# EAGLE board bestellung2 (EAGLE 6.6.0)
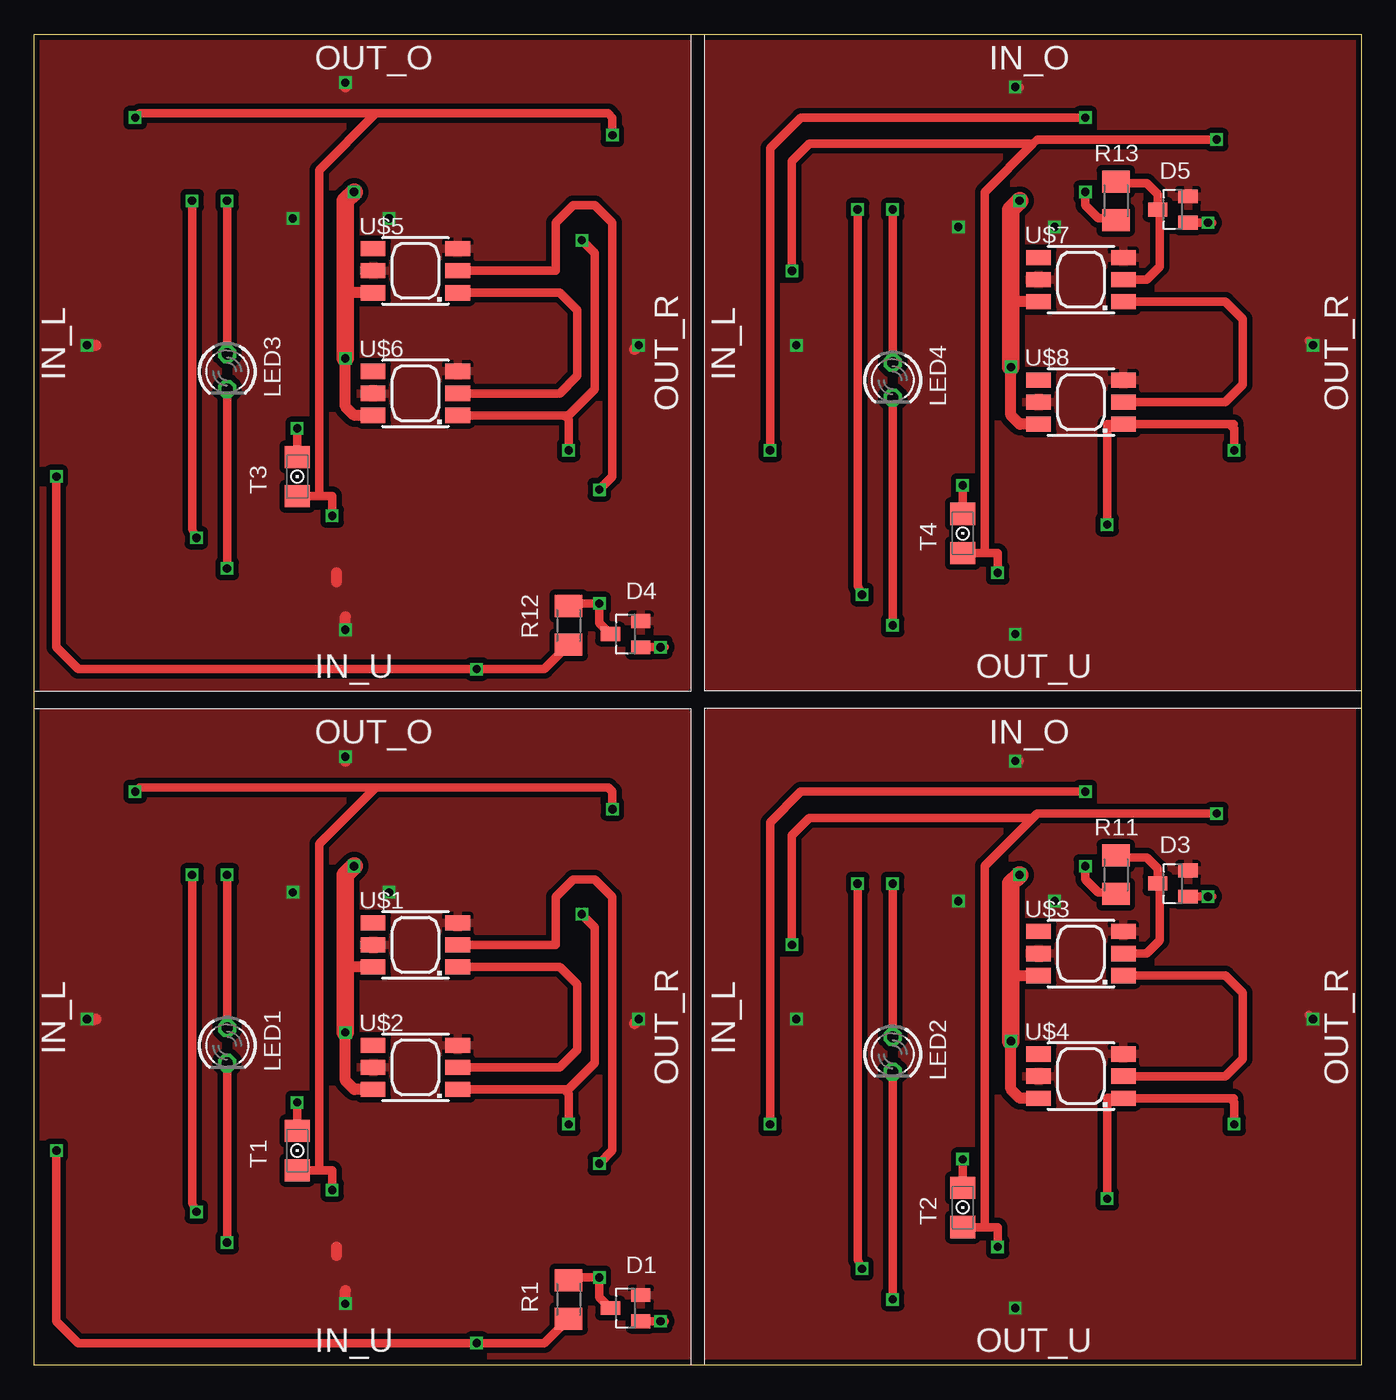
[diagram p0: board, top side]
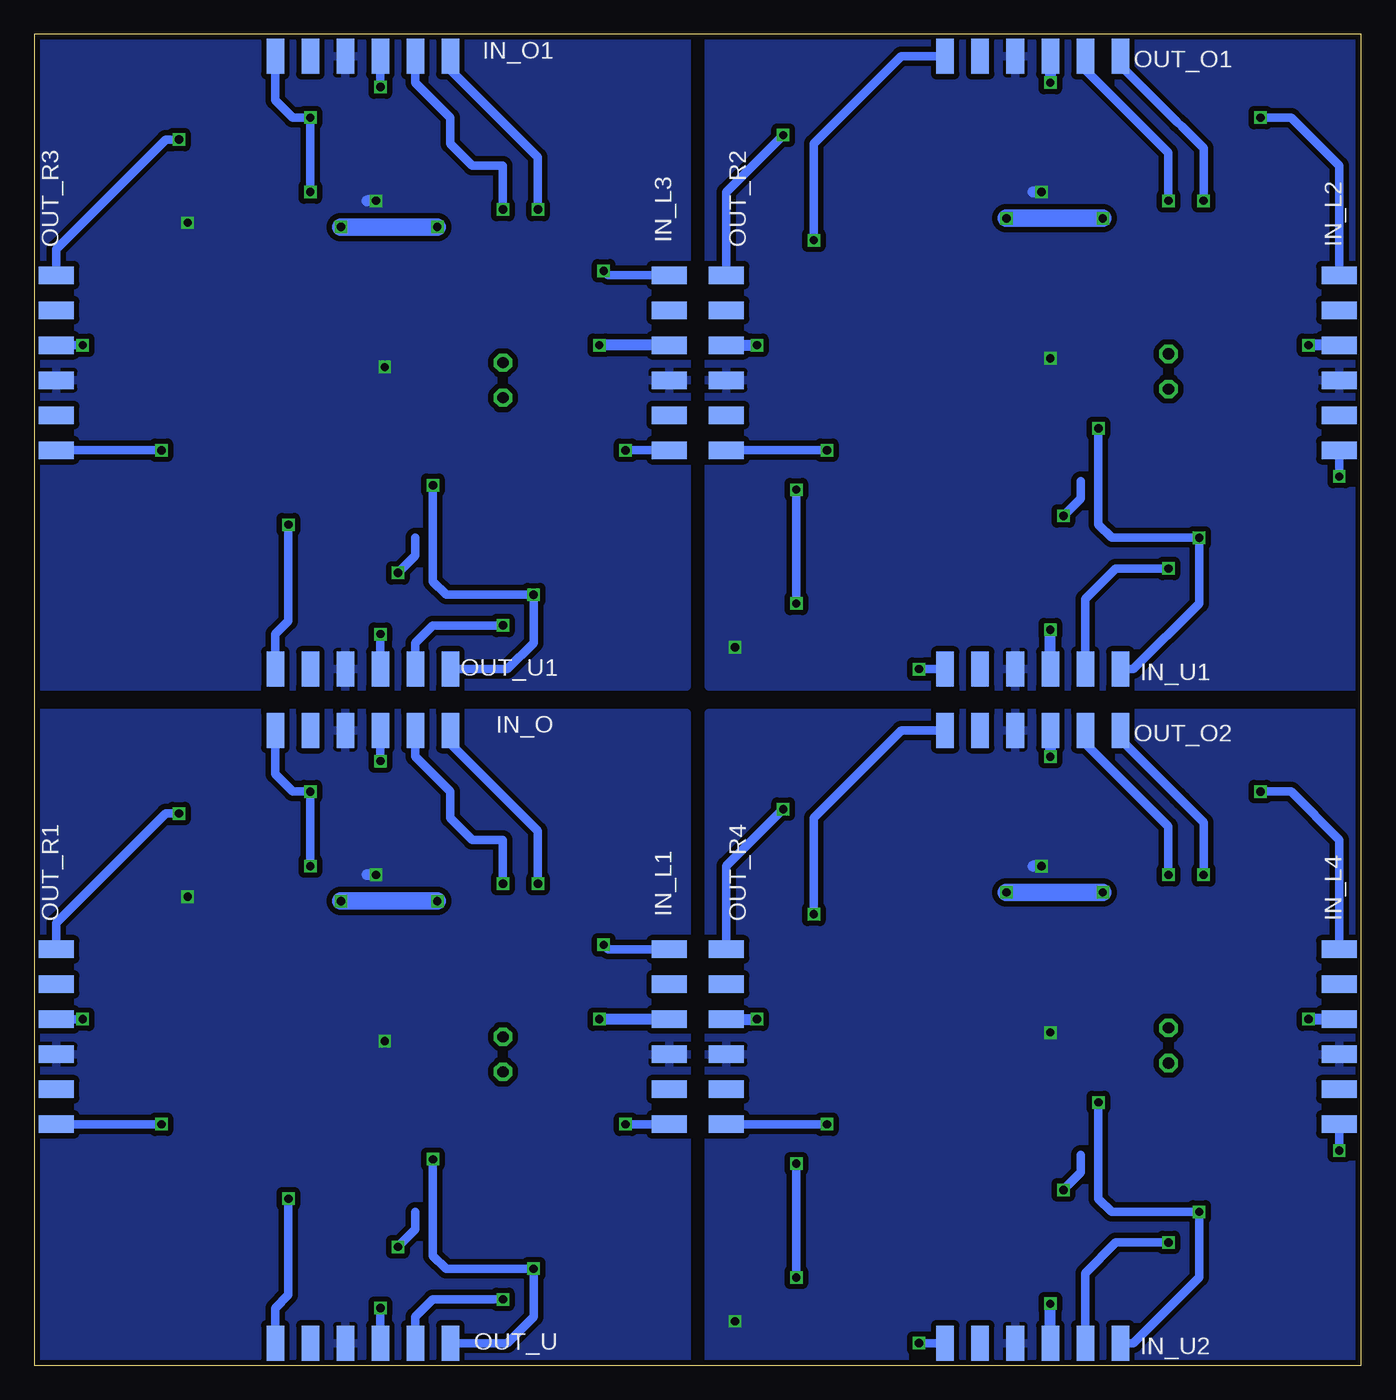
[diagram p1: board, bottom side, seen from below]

Size 96.2 x 96.52 mm. Coordinates in mm from the lower left corner, seen from the top.
Outline: 0,0 0,96.52 96.2,96.52 96.2,0 0,0
Copper layers (1*16): Top 0.035mm / dielectric 1.5mm / Bottom 0.035mm
Design rules "Elecrow_2-layer_eagle_rule": minimum track width 6mil, minimum drill 12mil, track to track 6mil, track to pad 6mil, pad to pad 6mil, via to via 6mil, smd to smd 0mil, copper to edge 10mil, drill to drill 10mil, minimum pad ring 10mil, minimum via ring 6mil, stop-mask expansion 2mil, vias tented up to drill 100mil, thermal gap 10mil

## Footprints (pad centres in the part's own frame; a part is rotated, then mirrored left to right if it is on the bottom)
SOT23 = smd 1 x 1.4: 1 -0.95,-1.1; 2 0.95,-1.1; 3 0,1.1
SMD1,27-2,54-6 = smd 1.27 x 2.54: 1 0,0; 2 2.54,0; 3 5.08,0; 4 7.62,0; 5 10.16,0; 6 12.7,0
LED3MM = drill 0.813 octagon: A -1.27,0; K 1.27,0
M1206 = smd 1.6 x 2: 1 -1.4,0; 2 1.4,0
1206 = smd 1.6 x 1.803: A -1.422,0; C 1.422,0
CLN6A = smd 1.778 x 1.1: 1 3.071,-1.6; 2 3.071,0; 3 3.071,1.6; 4 -3.071,1.6; 5 -3.071,0; 6 -3.071,-1.6

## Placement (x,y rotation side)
D1  BAS40-04  [SOT23]  42.86,4.13 90 top
D3  BAS40-04  [SOT23]  82.55,34.92 90 top
D4  BAS40-04  [SOT23]  42.86,53.02 90 top
D5  BAS40-04  [SOT23]  82.55,83.82 90 top
IN_L1  SMD2-6  [SMD1,27-2,54-6]  50.16,30.16 270 bottom
IN_L2  SMD2-6  [SMD1,27-2,54-6]  1.59,79.06 270 bottom
IN_L3  SMD2-6  [SMD1,27-2,54-6]  50.16,79.06 270 bottom
IN_L4  SMD2-6  [SMD1,27-2,54-6]  1.59,30.16 270 bottom
IN_O  SMD2-6  [SMD1,27-2,54-6]  66.04,46.04 180 bottom
IN_O1  SMD2-6  [SMD1,27-2,54-6]  66.04,94.93 180 bottom
IN_U1  SMD2-6  [SMD1,27-2,54-6]  17.46,50.48 180 bottom
IN_U2  SMD2-6  [SMD1,27-2,54-6]  17.46,1.59 180 bottom
LED1  [LED3MM]  13.97,23.18 270 top
LED2  [LED3MM]  62.23,22.54 270 top
LED3  [LED3MM]  13.97,72.07 270 top
LED4  [LED3MM]  62.23,71.44 270 top
OUT_O1  SMD2-6  [SMD1,27-2,54-6]  17.46,94.93 180 bottom
OUT_O2  SMD2-6  [SMD1,27-2,54-6]  17.46,46.04 180 bottom
OUT_R1  SMD2-6  [SMD1,27-2,54-6]  94.61,30.16 270 bottom
OUT_R2  SMD2-6  [SMD1,27-2,54-6]  46.04,79.06 270 bottom
OUT_R3  SMD2-6  [SMD1,27-2,54-6]  94.61,79.06 270 bottom
OUT_R4  SMD2-6  [SMD1,27-2,54-6]  46.04,30.16 270 bottom
OUT_U  SMD2-6  [SMD1,27-2,54-6]  66.04,1.59 180 bottom
OUT_U1  SMD2-6  [SMD1,27-2,54-6]  66.04,50.48 180 bottom
R1  [M1206]  38.73,4.76 90 top
R11  [M1206]  78.42,35.56 90 top
R12  [M1206]  38.73,53.66 90 top
R13  [M1206]  78.42,84.45 90 top
T1  PHOTO-TRANS-1206  [1206]  19.05,15.56 90 top
T2  PHOTO-TRANS-1206  [1206]  67.31,11.43 90 top
T3  PHOTO-TRANS-1206  [1206]  19.05,64.45 90 top
T4  PHOTO-TRANS-1206  [1206]  67.31,60.33 90 top
U$1  LED_SMD5050  [CLN6A]  27.62,30.48 0 top
U$2  LED_SMD5050  [CLN6A]  27.62,21.59 0 top
U$3  LED_SMD5050  [CLN6A]  75.88,29.84 0 top
U$4  LED_SMD5050  [CLN6A]  75.88,20.95 0 top
U$5  LED_SMD5050  [CLN6A]  27.62,79.38 0 top
U$6  LED_SMD5050  [CLN6A]  27.62,70.48 0 top
U$7  LED_SMD5050  [CLN6A]  75.88,78.74 0 top
U$8  LED_SMD5050  [CLN6A]  75.88,69.85 0 top

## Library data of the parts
D1 D3-D5 = diode
IN_L1-IN_L4 IN_O IN_O1 IN_U1 IN_U2 OUT_O1 OUT_O2 OUT_R1-OUT_R4 OUT_U OUT_U1 T1-T4 U$1-U$8 = #mylib
LED1-LED4 = led
R1 R11-R13 = resistor

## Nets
+5V1: D3.2 IN_L1.3 IN_O.3 OUT_R1.3 OUT_U.3 U$3.3 U$3.5 U$4.3 U$4.5
+5V2: D4.2 IN_L2.3 IN_U1.3 OUT_O1.3 OUT_R2.3 U$5.3 U$5.5 U$6.3 U$6.5
+5V3: D5.2 IN_L3.3 IN_O1.3 OUT_R3.3 OUT_U1.3 U$7.3 U$7.5 U$8.3 U$8.5
+5V4: D1.2 IN_L4.3 IN_U2.3 OUT_O2.3 OUT_R4.3 U$1.3 U$1.5 U$2.3 U$2.5
GND1: D3.1 IN_L1.4 IN_O.4 OUT_R1.4 OUT_U.4 U$3.6 U$4.6
GND2: D4.1 IN_L2.4 IN_U1.4 OUT_O1.4 OUT_R2.4 U$5.6 U$6.6
GND3: D5.1 IN_L3.4 IN_O1.4 OUT_R3.4 OUT_U1.4 U$7.6 U$8.6
GND4: D1.1 IN_L4.4 IN_U2.4 OUT_O2.4 OUT_R4.4 U$1.6 U$2.6
N$1: U$1.1 U$2.2
N$2: IN_U2.1 OUT_O2.1 T1.C
N$3: LED1.A OUT_O2.2
N$4: IN_U2.2 LED1.K
N$5: IN_L4.6 IN_U2.6 R1.1
N$6: IN_L4.1 OUT_R4.1 T1.A
N$7: D1.3 R1.2 U$1.2
N$8: OUT_O2.6 OUT_R4.6 U$2.1
N$12: U$3.1 U$4.2
N$16: IN_O.1 OUT_U.1 T2.C
N$20: IN_O.2 LED2.A
N$22: LED2.K OUT_U.2
N$23: IN_L1.6 IN_O.6 R11.1
N$24: IN_L1.1 OUT_R1.1 T2.A
N$26: D3.3 R11.2 U$3.2
N$27: OUT_R1.6 OUT_U.6 U$4.1
N$28: U$5.1 U$6.2
N$29: IN_U1.1 OUT_O1.1 T3.C
N$30: LED3.A OUT_O1.2
N$31: IN_U1.2 LED3.K
N$32: IN_L2.6 IN_U1.6 R12.1
N$33: IN_L2.1 OUT_R2.1 T3.A
N$34: D4.3 R12.2 U$5.2
N$35: OUT_O1.6 OUT_R2.6 U$6.1
N$36: U$7.1 U$8.2
N$37: IN_O1.1 OUT_U1.1 T4.C
N$38: IN_O1.2 LED4.A
N$39: LED4.K OUT_U1.2
N$40: IN_L3.6 IN_O1.6 R13.1
N$41: IN_L3.1 OUT_R3.1 T4.A
N$42: D5.3 R13.2 U$7.2
N$43: OUT_R3.6 OUT_U1.6 U$8.1

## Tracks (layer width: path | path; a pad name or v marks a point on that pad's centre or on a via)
+5V1  (via drill 0.6)
  Top 0.61: v71.12,43.81 71.44,43.81 | v92.71,25.08 92.39,25.4
  Bottom 0.61: IN_O.3 v71.12,43.81 | OUT_R1.3 v92.71,25.08 | v71.12,4.13 OUT_U.3
  Bottom 0.813: IN_L1.3 v55.24,25.08
  Bottom 1.27: v66.99,33.66 v73.98,33.66
  pour Top (isolate 0.406): 48.9,47.31 95.89,47.31 95.89,0.32 48.9,0.32
+5V2  (via drill 0.6)
  Top 0.813: 21.91,56.83 21.91,57.47 | v43.81,73.98 43.5,73.66 | v22.54,53.34 22.54,54.29 | v3.81,73.98 4.45,73.98 | v22.54,93.03 22.54,92.71
  Bottom 0.813: OUT_R2.3 v43.81,73.98 | IN_U1.3 v22.54,53.34 | IN_L2.3 v3.81,73.98 | OUT_O1.3 v22.54,93.03
  Bottom 1.27: v18.73,83.19 v25.72,83.19
  pour Top (isolate 0.406): 0.32,96.2 47.31,96.2 47.31,49.21 0.32,49.21
+5V3  (via drill 0.6)
  Top 0.61: v71.12,92.71 71.44,92.71 | v92.71,73.98 92.39,74.3
  Bottom 0.61: IN_O1.3 v71.12,92.71 | OUT_R3.3 v92.71,73.98 | v71.12,53.02 OUT_U1.3
  Bottom 0.813: IN_L3.3 v55.24,73.98
  Bottom 1.27: v66.99,82.55 v73.98,82.55
  pour Top (isolate 0.406): 48.9,96.2 95.89,96.2 95.89,49.21 48.9,49.21
+5V4  (via drill 0.6)
  Top 0.813: 21.91,7.94 21.91,8.57 | v43.81,25.08 43.5,24.77 | v22.54,4.45 22.54,5.4 | v3.81,25.08 4.45,25.08 | v22.54,44.13 22.54,43.81
  Bottom 0.813: OUT_R4.3 v43.81,25.08 | IN_U2.3 v22.54,4.45 | IN_L4.3 v3.81,25.08 | OUT_O2.3 v22.54,44.13
  Bottom 1.27: v18.73,34.29 v25.72,34.29
  pour Top (isolate 0.406): 0.32,47.31 47.31,47.31 47.31,0.32 0.32,0.32
GND1  (via drill 0.6)
  Top 0.61: D3.1 85.41,33.98 v85.09,33.97
  Top 0.813: U$4.6 71.45,19.36 70.8,20 v70.8,23.5 | U$3.6 70.81,28.25 70.8,28.26
  Top 1.27: v70.8,23.5 70.8,28.26 70.8,34.92 v71.44,35.56
  Bottom 0.813: v71.44,35.56 72.07,35.56
  pour Bottom (isolate 0.406): 48.9,47.31 95.89,47.31 95.89,0.32 48.9,0.32
GND2  (via drill 0.6)
  Top 0.61: D4.1 45.72,52.07 v45.4,52.07
  Top 0.813: U$6.6 23.19,68.89 22.54,69.53 v22.54,73.03 | U$5.6 22.55,77.78 22.54,77.79
  Top 1.27: v22.54,73.03 22.54,77.79 22.54,84.45 v23.18,85.09
  Bottom 0.813: v23.18,85.09 23.81,85.09
  pour Bottom (isolate 0.406): 0.32,96.2 47.31,96.2 47.31,49.21 0.32,49.21
GND3  (via drill 0.6)
  Top 0.61: D5.1 85.41,82.87 v85.09,82.87
  Top 0.813: U$8.6 71.45,68.25 70.8,68.9 v70.8,72.39 | U$7.6 70.81,77.14 70.8,77.15
  Top 1.27: v70.8,72.39 70.8,77.15 70.8,83.82 v71.44,84.45
  Bottom 0.813: v71.44,84.45 72.07,84.45
  pour Bottom (isolate 0.406): 48.9,96.2 95.89,96.2 95.89,49.21 48.9,49.21
GND4  (via drill 0.6)
  Top 0.61: D1.1 45.72,3.18 v45.4,3.17
  Top 0.813: U$2.6 23.19,19.99 22.54,20.64 v22.54,24.13 | U$1.6 22.55,28.88 22.54,28.89
  Top 1.27: v22.54,24.13 22.54,28.89 22.54,35.56 v23.18,36.2
  Bottom 0.813: v23.18,36.2 23.81,36.2
  pour Bottom (isolate 0.406): 0.32,47.31 47.31,47.31 47.31,0.32 0.32,0.32
N$1
  Top 0.61: U$2.2 38.1,21.59 39.37,22.86 39.37,27.62 38.1,28.89 30.71,28.89 U$1.1
N$2  (via drill 0.6)
  Top 0.61: v11.43,35.56 11.43,11.75 v11.75,11.11 | v19.05,19.05 T1.C
  Bottom 0.61: v11.43,35.56 11.43,39.37 13.02,40.96 13.34,41.27 17.46,45.4 OUT_O2.1 | v19.05,19.05 19.05,12.06 18.1,11.11 v11.75,11.11 11.75,6.35 16.51,1.59 IN_U2.1
N$3  (via drill 0.6)
  Top 0.61: v13.97,35.56 LED1.A
  Bottom 0.61: v13.97,35.56 13.97,39.05 20,45.09 OUT_O2.2
N$4  (via drill 0.6)
  Top 0.61: v13.97,8.89 LED1.K
  Bottom 0.61: v13.97,8.89 17.78,8.89 20,6.67 IN_U2.2
N$5  (via drill 0.6)
  Top 0.61: R1.1 36.96,1.59 v32.07,1.59 3.17,1.59 1.59,3.17 v1.59,15.56
  Bottom 0.61: IN_U2.6 v32.07,1.59 | IN_L4.6 v1.59,15.56
N$6  (via drill 0.6)
  Top 0.61: v21.59,12.7 21.59,14.14 T1.A 20.64,14.14 20.64,37.78 24.77,41.91 | v41.91,40.32 41.91,41.59 41.59,41.91 24.77,41.91 | v7.3,41.59 7.62,41.91 24.77,41.91
  Bottom 0.61: 20.32,15.24 20.32,13.97 v21.59,12.7 | OUT_R4.1 46.04,36.2 v41.91,40.32 | v7.3,41.59 5.08,41.59 1.59,38.1 IN_L4.1
N$7  (via drill 0.6)
  Top 0.61: 41.91,3.98 D1.3 40.96,4.93 v40.96,6.35 38.92,6.35 R1.2 | U$1.2 37.78,30.48 37.78,33.97 39.05,35.24 40.64,35.24 41.91,33.97 41.91,15.56 v40.96,14.61
  Bottom 0.61: v40.96,6.35 v40.96,14.61
N$8  (via drill 0.6)
  Top 0.61: U$2.1 38.42,19.99 | 38.42,19.99 38.72,19.99 40.64,21.91 40.64,31.75 v39.69,32.7 | v38.73,17.46 38.73,19.67 38.42,19.99
  Bottom 0.61: v39.69,32.7 39.69,39.69 33.34,46.04 OUT_O2.6 | OUT_R4.6 v38.73,17.46
N$12
  Top 0.61: U$4.2 86.36,20.95 87.63,22.23 87.63,26.99 86.36,28.26 78.97,28.26 U$3.1
N$16  (via drill 0.6)
  Top 0.61: v59.69,34.92 59.69,7.62 v60.01,6.99 | v67.31,14.92 T2.C
  Bottom 0.61: v59.69,34.92 59.69,38.73 66.04,45.09 IN_O.1 | v67.31,14.92 67.31,7.94 66.36,6.99 v60.01,6.99 60.01,3.49 61.91,1.59 OUT_U.1
N$20  (via drill 0.6)
  Top 0.61: v62.23,34.92 LED2.A
  Bottom 0.61: v62.23,34.92 62.23,38.1 64.45,38.1 66.04,39.69 66.04,41.59 68.58,44.13 IN_O.2
N$22  (via drill 0.6)
  Top 0.61: v62.23,4.76 LED2.K
  Bottom 0.61: OUT_U.2 68.58,3.49 67.31,4.76 v62.23,4.76
N$23  (via drill 0.6)
  Top 0.61: v76.2,36.2 76.2,35.24 77.15,34.29 78.29,34.29 R11.1 | v53.34,17.46 53.34,39.37 55.56,41.59 v76.2,41.59
  Bottom 0.61: v76.2,36.2 v76.2,41.59 77.47,41.59 78.74,42.86 IN_O.6 | IN_L1.6 v53.34,17.46
N$24  (via drill 0.6)
  Top 0.61: v69.85,8.57 69.85,10.01 68.9,10.01 | 72.39,39.69 72.71,40.01 v85.72,40.01 | 72.39,39.69 68.9,36.2 68.9,10.01 | 68.9,10.01 T2.A | v54.93,30.48 54.93,38.42 56.2,39.69 72.39,39.69
  Bottom 0.61: 68.58,11.11 68.58,9.84 v69.85,8.57 | v85.72,40.01 86.68,40.01 94.61,32.07 OUT_R1.1 | IN_L1.1 54.61,30.16 v54.93,30.48
N$26
  Top 0.61: U$3.2 80.64,29.84 81.6,30.8 81.6,34.78 D3.3 81.45,36.02 80.64,36.83 78.55,36.83 R11.2
N$27  (via drill 0.6)
  Top 0.61: 86.68,19.36 U$4.1 78.95,19.37 77.79,19.37 v77.79,12.06 | 86.68,19.36 86.98,19.36 | v87,17.46 87,19.04 86.68,19.36
  Bottom 0.61: OUT_R1.6 v87,17.46 | v77.79,12.06 77.79,5.08 78.74,4.13 OUT_U.6
N$28
  Top 0.61: U$6.2 38.1,70.48 39.37,71.75 39.37,76.52 38.1,77.79 30.71,77.79 U$5.1
N$29  (via drill 0.6)
  Top 0.61: v11.43,84.45 11.43,60.64 v11.75,60.01 | v19.05,67.94 T3.C
  Bottom 0.61: v11.43,84.45 11.43,88.27 13.02,89.85 13.34,90.17 17.46,94.3 OUT_O1.1 | v19.05,67.94 19.05,60.96 18.1,60.01 v11.75,60.01 11.75,55.24 16.51,50.48 IN_U1.1
N$30  (via drill 0.6)
  Top 0.61: v13.97,84.45 LED3.A
  Bottom 0.61: v13.97,84.45 13.97,87.95 20,93.98 OUT_O1.2
N$31  (via drill 0.6)
  Top 0.61: v13.97,57.78 LED3.K
  Bottom 0.61: v13.97,57.78 17.78,57.78 20,55.56 IN_U1.2
N$32  (via drill 0.6)
  Top 0.61: R12.1 36.96,50.48 v32.07,50.48 3.17,50.48 1.59,52.07 v1.59,64.45
  Bottom 0.61: IN_U1.6 v32.07,50.48 | IN_L2.6 v1.59,64.45
N$33  (via drill 0.6)
  Top 0.61: v21.59,61.59 21.59,63.03 T3.A 20.64,63.03 20.64,86.68 24.77,90.81 | v41.91,89.22 41.91,90.49 41.59,90.81 24.77,90.81 | v7.3,90.49 7.62,90.81 24.77,90.81
  Bottom 0.61: 20.32,64.14 20.32,62.87 v21.59,61.59 | OUT_R2.1 46.04,85.09 v41.91,89.22 | v7.3,90.49 5.08,90.49 1.59,87 IN_L2.1
N$34  (via drill 0.6)
  Top 0.61: 41.91,52.88 D4.3 40.96,53.83 v40.96,55.24 38.92,55.24 R12.2 | U$5.2 37.78,79.38 37.78,82.87 39.05,84.14 40.64,84.14 41.91,82.87 41.91,64.45 v40.96,63.5
  Bottom 0.61: v40.96,55.24 v40.96,63.5
N$35  (via drill 0.6)
  Top 0.61: U$6.1 38.42,68.89 | 38.42,68.89 38.72,68.89 40.64,70.8 40.64,80.64 v39.69,81.6 | v38.73,66.36 38.73,68.57 38.42,68.89
  Bottom 0.61: v39.69,81.6 39.69,88.58 33.34,94.93 OUT_O1.6 | OUT_R2.6 v38.73,66.36
N$36
  Top 0.61: U$8.2 86.36,69.85 87.63,71.12 87.63,75.88 86.36,77.15 78.97,77.15 U$7.1
N$37  (via drill 0.6)
  Top 0.61: v59.69,83.82 59.69,56.52 v60.01,55.88 | v67.31,63.82 T4.C
  Bottom 0.61: v59.69,83.82 59.69,87.63 66.04,93.98 IN_O1.1 | v67.31,63.82 67.31,56.83 66.36,55.88 v60.01,55.88 60.01,52.39 61.91,50.48 OUT_U1.1
N$38  (via drill 0.6)
  Top 0.61: v62.23,83.82 LED4.A
  Bottom 0.61: v62.23,83.82 62.23,87 64.45,87 66.04,88.58 66.04,90.49 68.58,93.03 IN_O1.2
N$39  (via drill 0.6)
  Top 0.61: v62.23,53.66 LED4.K
  Bottom 0.61: OUT_U1.2 68.58,52.39 67.31,53.66 v62.23,53.66
N$40  (via drill 0.6)
  Top 0.61: v76.2,85.09 76.2,84.14 77.15,83.19 78.29,83.19 R13.1 | v53.34,66.36 53.34,88.27 55.56,90.49 v76.2,90.49
  Bottom 0.61: v76.2,85.09 v76.2,90.49 77.47,90.49 78.74,91.76 IN_O1.6 | IN_L3.6 v53.34,66.36
N$41  (via drill 0.6)
  Top 0.61: v69.85,57.47 69.85,58.9 68.9,58.9 | 72.39,88.58 72.71,88.9 v85.72,88.9 | 72.39,88.58 68.9,85.09 68.9,58.9 | 68.9,58.9 T4.A | v54.93,79.38 54.93,87.31 56.2,88.58 72.39,88.58
  Bottom 0.61: 68.58,60.01 68.58,58.74 v69.85,57.47 | v85.72,88.9 86.68,88.9 94.61,80.96 OUT_R3.1 | IN_L3.1 54.61,79.06 v54.93,79.38
N$42
  Top 0.61: U$7.2 80.64,78.74 81.6,79.69 81.6,83.67 D5.3 81.45,84.92 80.64,85.72 78.55,85.72 R13.2
N$43  (via drill 0.6)
  Top 0.61: 86.68,68.25 U$8.1 78.95,68.26 77.79,68.26 v77.79,60.96 | 86.68,68.25 86.98,68.25 | v87,66.36 87,67.93 86.68,68.25
  Bottom 0.61: OUT_R3.6 v87,66.36 | v77.79,60.96 77.79,53.98 78.74,53.02 OUT_U1.6

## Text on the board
tNames: OUT_O | IN_O | IN_L | IN_L | OUT_R | OUT_R | IN_U | OUT_U | OUT_O | IN_O | IN_L | IN_L | OUT_R | OUT_R | IN_U | OUT_U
